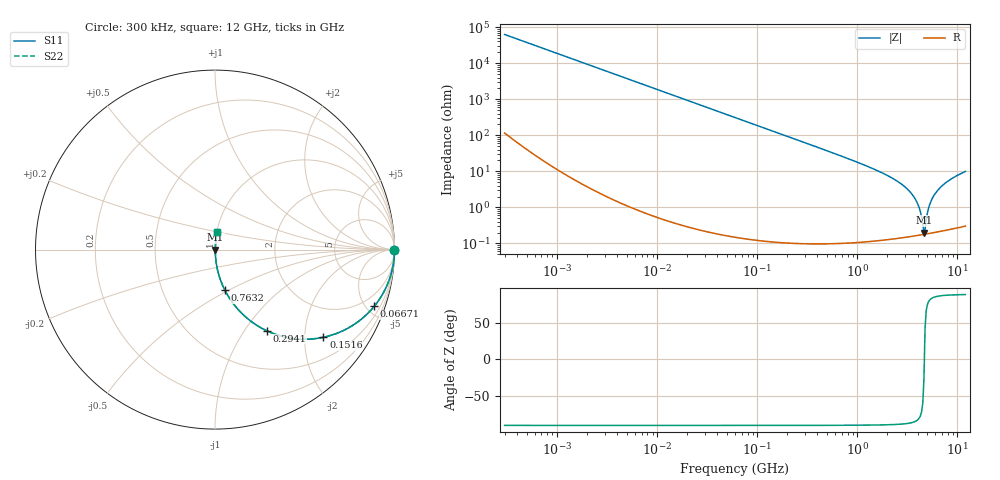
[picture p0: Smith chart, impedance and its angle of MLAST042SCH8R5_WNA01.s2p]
! MLAST042SCH8R5_WNA01  S-PARAMETER MODEL  ( General Type )
! Model Generated by TAIYO YUDEN Corporation (http://www.ty-top.com)
! Version 1.0
! TAIYO YUDEN Control No. 150820
! Copyright(c) 2015 TAIYO YUDEN CO.,LTD. All Rights Reserved.
! Product Description (link to TY-COMPAS)
! https://ds.yuden.co.jp/TYCOMPAS/or/detail?pn=MLAST042SCH8R5BWNA01&u=M
! Products Name : Multilayer Ceramic Capacitors
! Characteristics :
!  Capacitance : 8.5 pF , Rated Voltage : 25V , TCC : CH / C0H
!  Case Size : 0.4 x 0.2 / 0.016 x 0.008 [mm/inch] , Thickness : 0.2 / 0.008 [mm/inch]
!  (Conditions: Temperature = 25 degC , DC Bias Current/Voltage = 0A / 0V)
! External Node Assignments :
!  1  o---| |---o  2
! GND o---------o GND
! Frequency Range : 0.3MHz  -  12000MHz  [ 401 STEP ]
# MHz S RI R 50
! Freq[MHz].  S11 Real  S11 Imag  S21 Real  S21 Imag  S12 Real  S12 Imag  S22 Real  S22 Imag
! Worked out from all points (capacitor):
!   401 points, 300 kHz to 12 GHz, reference 50 ohm
!   read as one part in series: C = 8.49 pF near 316.3 kHz
!   lowest |Z| = 201 mohm at 4.624 GHz (marker M1)
!   series resonance near 4.668 GHz, so ESL is about 140 pH
!   S11 on the Smith chart (normalised r, x): 300 kHz: open; 66.71 MHz: 1.00, -5.62; 151.6 MHz: 1.00, -2.47; 294.1 MHz: 1.00, -1.27; 763.2 MHz: 1.00, -0.48; 12 GHz: 1.01, +0.20
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0.3  1 -0.0016  5.51e-06 0.0016  5.51e-06 0.0016  1 -0.0016
1.769972  0.9999 -0.00944  9.31e-05 0.00944  9.31e-05 0.00944  0.9999 -0.00944
10.44266  0.9969 -0.0555  0.00311 0.0555  0.00311 0.0555  0.9969 -0.0555
26.39317  0.9805 -0.138  0.0195 0.138  0.0195 0.138  0.9805 -0.138
60  0.9069 -0.2903  0.0931 0.2903  0.0931 0.2903  0.9069 -0.2903
66.70707  0.8874 -0.3158  0.1126 0.3158  0.1126 0.3158  0.8874 -0.3158
151.6462  0.6039 -0.4887  0.3961 0.4887  0.3961 0.4887  0.6039 -0.4887
294.0765  0.2876 -0.4519  0.7124 0.4519  0.7124 0.4519  0.2876 -0.4519
353.9943  0.2175 -0.4116  0.7825 0.4116  0.7825 0.4116  0.2175 -0.4116
763.2128  0.0549 -0.2257  0.9451 0.2257  0.9451 0.2257  0.0549 -0.2257
2088.533  0.00641 -0.0713  0.9936 0.0713  0.9936 0.0713  0.00641 -0.0713
2870.14  0.00309 -0.0405  0.9969 0.0405  0.9969 0.0405  0.00309 -0.0405
3547.679  0.00208 -0.0223  0.9979 0.0223  0.9979 0.0223  0.00208 -0.0223
4050.141  0.00181 -0.0115  0.9982 0.0115  0.9982 0.0115  0.00181 -0.0115
4502.883  0.00177 -0.003  0.9982 0.003  0.9982 0.003  0.00177 -0.003
4623.766  0.00178 -0.000931  0.9982 0.000931  0.9982 0.000931  0.00178 -0.000931
4875.354  0.00184 0.00421  0.9982 -0.00421  0.9982 -0.00421  0.00184 0.00421
5140.631  0.00196 0.00927  0.998 -0.00927  0.998 -0.00927  0.00196 0.00927
5420.343  0.00213 0.0143  0.9979 -0.0143  0.9979 -0.0143  0.00213 0.0143
6188.031  0.0028 0.0271  0.9972 -0.0271  0.9972 -0.0271  0.0028 0.0271
8064.993  0.00529 0.0538  0.9947 -0.0538  0.9947 -0.0538  0.00529 0.0538
12000  0.0127 0.0979  0.9873 -0.0979  0.9873 -0.0979  0.0127 0.0979
